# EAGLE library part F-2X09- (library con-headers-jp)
FEMALE HEADER
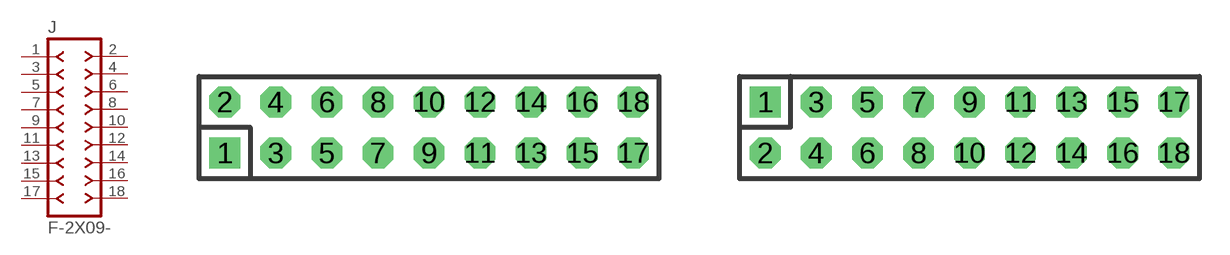
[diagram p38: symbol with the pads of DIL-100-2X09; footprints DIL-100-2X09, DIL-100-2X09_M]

Designator prefix J

## F-2X09-DIL-100  [DIL-100-2X09]
1  1  pas
2  2  pas
3  3  pas
4  4  pas
5  5  pas
6  6  pas
7  7  pas
8  8  pas
9  9  pas
10  10  pas
11  11  pas
12  12  pas
13  13  pas
14  14  pas
15  15  pas
16  16  pas
17  17  pas
18  18  pas

## F-2X09-DIL-100_M  [DIL-100-2X09_M]
Pads as for DIL-100-2X09

## F-2X09-DIL-2MM  [DIL-2MM-2X09]
Pads as for DIL-100-2X09

## F-2X09-DIL-2MM_M  [DIL-2MM-2X09_M]
Pads as for DIL-100-2X09

## F-2X09-71991  [71991-18]
Pads as for DIL-100-2X09

## F-2X09-79107  [79107-18]
Pads as for DIL-100-2X09

## F-2X09-79107_M  [79107-18_M]
Pads as for DIL-100-2X09

## Footprint DIL-100-2X09 (pad centres in mm)
PIN HEADER - 0.1"
drill 1.016 square: 1 -10.16,-1.27
drill 1.016 octagon: 2 -10.16,1.27; 3 -7.62,-1.27; 4 -7.62,1.27; 5 -5.08,-1.27; 6 -5.08,1.27; 7 -2.54,-1.27; 8 -2.54,1.27; 9 0,-1.27; 10 0,1.27; 11 2.54,-1.27; 12 2.54,1.27; 13 5.08,-1.27; 14 5.08,1.27; 15 7.62,-1.27; 16 7.62,1.27; 17 10.16,-1.27; 18 10.16,1.27

## Footprint DIL-100-2X09_M (pad centres in mm)
PIN HEADER - MIRRORED 0.1"
drill 1.016 square: 1 -10.16,1.27
drill 1.016 octagon: 2 -10.16,-1.27; 3 -7.62,1.27; 4 -7.62,-1.27; 5 -5.08,1.27; 6 -5.08,-1.27; 7 -2.54,1.27; 8 -2.54,-1.27; 9 0,1.27; 10 0,-1.27; 11 2.54,1.27; 12 2.54,-1.27; 13 5.08,1.27; 14 5.08,-1.27; 15 7.62,1.27; 16 7.62,-1.27; 17 10.16,1.27; 18 10.16,-1.27

## Footprint DIL-2MM-2X09 (pad centres in mm)
PIN HEADER - 2MM"
drill 0.711 square: 1 -8,-1
drill 0.711: 2 -8,1; 3 -6,-1; 4 -6,1; 5 -4,-1; 6 -4,1; 7 -2,-1; 8 -2,1; 9 0,-1; 10 0,1; 11 2,-1; 12 2,1; 13 4,-1; 14 4,1; 15 6,-1; 16 6,1; 17 8,-1; 18 8,1

## Footprint DIL-2MM-2X09_M (pad centres in mm)
PIN HEADER - MIRRORED 2MM
drill 0.711 square: 1 -8,1
drill 0.711: 2 -8,-1; 3 -6,1; 4 -6,-1; 5 -4,1; 6 -4,-1; 7 -2,1; 8 -2,-1; 9 0,1; 10 0,-1; 11 2,1; 12 2,-1; 13 4,1; 14 4,-1; 15 6,1; 16 6,-1; 17 8,1; 18 8,-1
